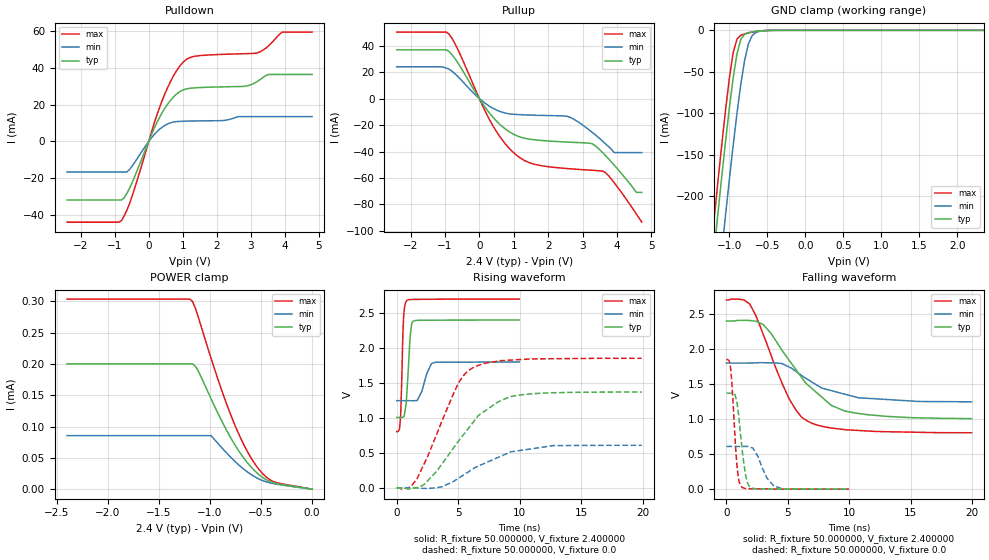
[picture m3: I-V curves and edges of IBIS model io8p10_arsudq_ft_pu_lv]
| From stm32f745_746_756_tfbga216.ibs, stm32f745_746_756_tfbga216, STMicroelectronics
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|   Model io8p10_arsudq_ft_pu_lv
[Model]  io8p10_arsudq_ft_pu_lv
Model_type I/O
Polarity   Non-Inverting
Enable   Active-Low
Vinl =   0.720000V
Vinh =   1.680000V
Vmeas =  1.200000V
Cref =   40.000000pF
Rref =   100.000000M
Vref =   0.0V
C_comp   2.239000pF   2.178700pF   2.334000pF
[Temperature Range]   25.000000   0.125000k   -40.000000
[Pullup Reference]   2.400000V   1.800000V   2.700000V
[Pulldown Reference]   0.0V   0.0V   0.0V
[POWER Clamp Reference]   2.400000V   1.800000V   2.700000V
[GND Clamp Reference]   0.0V   0.0V   0.0V
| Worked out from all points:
|   slope of the pulldown table from 0 to 0.36 V, typ, clamps not added: 25 ohm
|   slope of the pullup table from 0 to 0.36 V, typ, clamps not added: 27.7 ohm
|   GND clamp passes 1 mA (typ) near -0.62 V on its own axis
|   rising waveform, R_fixture 50.000000, V_fixture 2.400000: 20-80 % time 276ps typ, 615ps min, 182ps max; typ from 1.01 V to 2.4 V
|   rising waveform, R_fixture 50.000000, V_fixture 0.0: 20-80 % time 3.74ns typ, 4.04ns min, 2.67ns max; typ from 0.001 V to 1.37 V
|   falling waveform, R_fixture 50.000000, V_fixture 2.400000: 20-80 % time 3.94ns typ, 4ns min, 2.72ns max; typ from 2.4 V to 1.01 V
|   falling waveform, R_fixture 50.000000, V_fixture 0.0: 20-80 % time 530ps typ, 980ps min, 384ps max; typ from 1.37 V to 0.001 V
[Pulldown]
|Voltage   I(typ)   I(min)   I(max)
-2.4V     -31.73mA   -16.51mA   -43.74mA
-800mV    -31.73mA   -16.51mA   -42.87mA
-480mV    -21.98mA   -13.17mA   -29.21mA
80mV      3.63mA     1.966mA    5.014mA
480mV     18.16mA    8.738mA    26.02mA
800mV     25.38mA    10.72mA    37.77mA
1.12V     28.53mA    11.02mA    44.6mA
2.8V      29.84mA    13.46mA    47.53mA
3.2V      32.6mA     13.46mA    48.03mA
3.52V     36.28mA    13.46mA    51.75mA
3.92V     36.28mA    13.46mA    59.24mA
4.8V      36.28mA    13.46mA    59.24mA
[Pullup]
|Voltage   I(typ)   I(min)   I(max)
-2.4V     36.81mA    24.03mA    50.22mA
-960mV    36.81mA    23mA       50.22mA
-640mV    27.63mA    17.02mA    37.96mA
320mV     -11.75mA   -6.207mA   -17.08mA
960mV     -26.47mA   -11.82mA   -40.02mA
1.52V     -30.88mA   -12.51mA   -49.05mA
2.56V     -32.88mA   -13.48mA   -52.9mA
3.28V     -34.18mA   -25.52mA   -54.17mA
3.6V      -41.3mA    -32.61mA   -54.97mA
3.92V     -50.32mA   -40.8mA    -63.62mA
4.56V     -70.9mA    -40.8mA    -87.07mA
4.72V     -70.9mA    -40.8mA    -93.4mA
[GND_clamp]
|Voltage   I(typ)   I(min)   I(max)
-2.4V     -1.424A    -1.508A    -1.393A
-1.25V    -311.2mA   -401.9mA   -273.3mA
-1.2V     -265.4mA   -356.1mA   -227.2mA
-1.15V    -220.4mA   -310.8mA   -181.9mA
-1.1V     -176.3mA   -266.2mA   -137.9mA
-1.05V    -133.8mA   -222.5mA   -95.87mA
-950mV    -57.3mA    -138.9mA   -26.98mA
-900mV    -28.27mA   -100.4mA   -10.59mA
-850mV    -11.01mA   -65.54mA   -5.958mA
-750mV    -2.834mA   -16.5mA    -3.178mA
-600mV    -750uA     -1.164mA   -738.3uA
2.35V     0A         0A         0A
[POWER_clamp]
|Voltage   I(typ)   I(min)   I(max)
-2.4V     200uA      85.39uA    303.5uA
-1.2V     200uA      85.39uA    303.5uA
-1.17V    200uA      85.39uA    299.5uA
-1.14V    195.7uA    85.39uA    287.5uA
-990mV    144.6uA    85.39uA    209.3uA
-870mV    104.1uA    63.61uA    150.8uA
-780mV    77.28uA    48.2uA     111.8uA
-660mV    47.71uA    30.75uA    68.21uA
-570mV    30.64uA    20.61uA    42.79uA
-480mV    18.19uA    13.44uA    24.07uA
-390mV    10.91uA    9.231uA    13.01uA
0V        0A         0A         0A
[Ramp]
| variable   typ   min   max
dV/dt_r  0.82207/3.74174n   0.36620/4.04163n   1.11383/2.67718n
dV/dt_f  0.83280/3.94394n   0.33222/4.06778n   1.13593/2.72612n
R_load = 50.000000
[Rising Waveform]
R_fixture= 50.000000
V_fixture= 2.400000
V_fixture_min= 1.800000
V_fixture_max= 2.700000
|time   V(typ)   V(min)   V(max)
0s        1.007V     1.247V     805.7mV
220.2ps   1.007V     1.247V     832.5mV
300.3ps   1.007V     1.247V     991.5mV
560.6ps   1.016V     1.247V     2.443V
820.8ps   1.349V     1.247V     2.677V
1.081ns   2.141V     1.247V     2.693V
1.341ns   2.383V     1.246V     2.694V
2.042ns   2.396V     1.381V     2.695V
2.843ns   2.397V     1.779V     2.697V
9.97ns    2.4V       1.8V       2.699V
[Rising Waveform]
R_fixture= 50.000000
V_fixture= 0.0
V_fixture_min= 0.0
V_fixture_max= 0.0
|time   V(typ)   V(min)   V(max)
0s        1.049mV    906.1uV    1.497mV
1.121ns   -12.38mV   964.5uV    16.25mV
1.642ns   3.5mV      328.2uV    126.3mV
3.283ns   245.8mV    4.465mV    783.5mV
4.965ns   655.6mV    132.2mV    1.479V
6.206ns   936.4mV    273mV      1.719V
8.168ns   1.222V     430.8mV    1.811V
9.57ns    1.315V     524.1mV    1.83V
12.77ns   1.361V     605.4mV    1.847V
19.94ns   1.371V     610.2mV    1.852V
[Falling Waveform]
R_fixture= 50.000000
V_fixture= 2.400000
V_fixture_min= 1.800000
V_fixture_max= 2.700000
|time   V(typ)   V(min)   V(max)
0s        2.4V       1.8V       2.699V
1.121ns   2.41V      1.8V       2.71V
1.882ns   2.407V     1.801V     2.645V
3.003ns   2.348V     1.805V     2.205V
5.085ns   1.844V     1.745V     1.295V
6.046ns   1.612V     1.632V     1.041V
6.767ns   1.466V     1.55V      956.4mV
8.529ns   1.197V     1.407V     873.6mV
9.89ns    1.107V     1.344V     847.2mV
19.94ns   1.007V     1.247V     805.7mV
[Falling Waveform]
R_fixture= 50.000000
V_fixture= 0.0
V_fixture_min= 0.0
V_fixture_max= 0.0
|time   V(typ)   V(min)   V(max)
0s        1.371V     610.2mV    1.852V
340.3ps   1.371V     610.2mV    1.721V
440.4ps   1.371V     610.2mV    1.523V
700.7ps   1.346V     610.1mV    730.1mV
940.9ps   1.128V     609.9mV    201.5mV
1.241ns   625.3mV    609.7mV    34.38mV
1.682ns   107.8mV    611.4mV    8.744mV
2.042ns   19.6mV     592.5mV    6.441mV
3.844ns   3.259mV    50.2mV     3.173mV
9.97ns    1.049mV    906.1uV    1.497mV
